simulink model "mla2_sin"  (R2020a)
settings: Solver=ode5  StartTime=0.0  StopTime=10  FixedStep=0.0001  RelTol=1e-4  EnableMultiTasking=on
PreLoadFcn:
  | MLA_Sensor1 = load('mla_sensor1.dat');
libraries: libmla x1

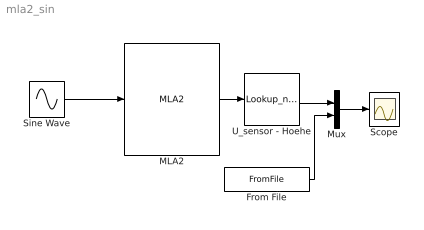
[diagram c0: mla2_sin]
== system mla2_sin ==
  From File : FromFile  FileName=mla_sin.mat  SampleTime=0
  MLA2 : libmla/MLA2  g=9.81  m=0.125  Fr_g=0.14  Fr_h=0.16  d_l=0.18  d_t=0.1  a=40691  b=0.0687  N=4.282
  Mux : Mux  Inputs=2
  Scope : Scope
  Sine Wave : Sin  Bias=2.5  Frequency=2  SampleTime=0
  U_sensor - Hoehe : Lookup_n-D  NumberOfTableDimensions=1  BreakpointsForDimension1=MLA_Sensor1(:,1)  Table=MLA_Sensor1(:,2)  RndMeth=Simplest
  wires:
  MLA2/1 -> U_sensor - Hoehe/1
  Sine Wave/1 -> MLA2/1
  U_sensor - Hoehe/1 -> Mux/1
  Mux/1 -> Scope/1
  From File/1 -> Mux/2
